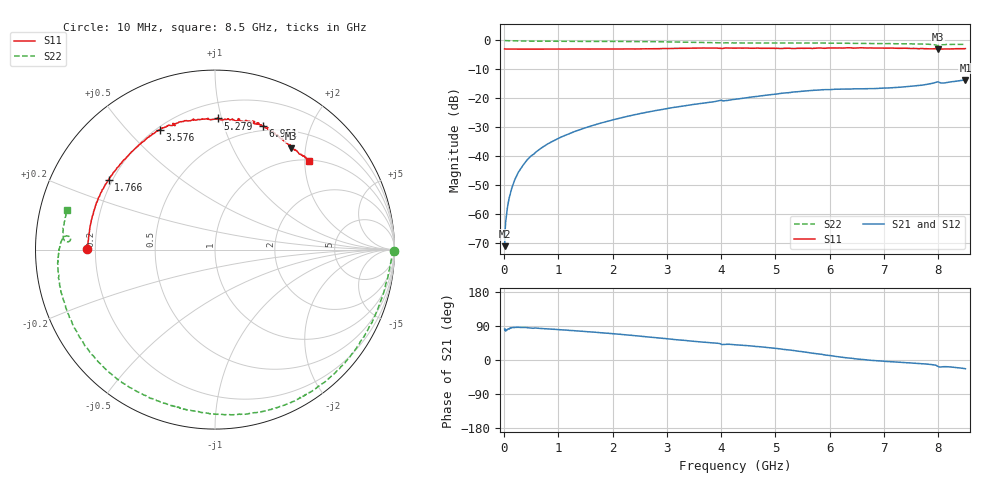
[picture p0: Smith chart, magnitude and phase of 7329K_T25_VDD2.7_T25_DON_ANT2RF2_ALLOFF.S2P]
!Agilent Technologies,E5071C,MY46417908,A.11.23
!Date: Mon Aug 31 18:03:31 2020
!Data & Calibration Information:
!Freq	S11:SOLT2(ON)	S21:SOLT2(ON)	S12:SOLT2(ON)	S22:SOLT2(ON)
!PortZ  Port1:50+j0  Port2:50+j0
!Above PortZ is port z conversion or system Z0 setting when saving the data.
!When reading, reference impedance value at option line is always used.
# Hz S dB R 50
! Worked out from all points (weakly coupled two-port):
!   1601 points, 10 MHz to 8.5 GHz, reference 50 ohm
!   highest |S21| = -13.61 dB at 8.5 GHz (marker M1); lowest = -71.0 dB at 10 MHz (marker M2)
!   lowest |S11| = -3.0 dB at 8.001 GHz (marker M3), VSWR 5.81, Z = 38.5 + j86.8 ohm
!   |S11| at or under -10 dB: nowhere
!   |S22| runs from -1.9 to 0.0 dB; largest |S21 - S12| = 0.003
!   S11 on the Smith chart (normalised r, x): 10 MHz: 0.17, +0.00; 1.766 GHz: 0.18, +0.29; 3.576 GHz: 0.21, +0.62; 5.279 GHz: 0.31, +0.97; 6.951 GHz: 0.45, +1.36; 8.5 GHz: 1.01, +2.10
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1e7  -2.95 179.8  -70.96 81.3  -70.53 82.9  -0.02 -0.4
6.836875e7  -2.99 178.5  -56.87 80.8  -57.05 80.9  -0.11 -2.0
1.214312e8  -2.99 177.3  -52.25 84.5  -52.21 84.3  -0.14 -3.3
2.169438e8  -3.01 175.3  -47.32 85.9  -47.27 86.3  -0.18 -5.3
3.389875e8  -3.01 173.0  -43.32 85.9  -43.29 86.2  -0.22 -8.1
4.822562e8  -3.01 170.1  -40.14 84.3  -40.15 84.5  -0.26 -11.4
7.634875e8  -3.00 164.8  -36.19 82.5  -36.19 82.5  -0.30 -17.7
1.426769e9  -2.98 152.8  -30.60 75.9  -30.58 75.9  -0.36 -33.4
1.766369e9  -2.98 146.6  -28.60 72.2  -28.59 72.2  -0.36 -41.4
2.843538e9  -2.85 126.1  -24.04 58.3  -24.04 58.2  -0.46 -67.0
3.5758e9  -2.66 114.8  -21.89 48.2  -21.88 48.3  -0.70 -86.0
4.255e9  -2.64 105.7  -20.33 40.2  -20.33 40.2  -0.88 -101.8
4.828075e9  -2.75 96.3  -18.90 33.2  -18.89 33.2  -0.90 -114.1
5.279106e9  -2.72 88.8  -17.96 26.2  -17.94 26.4  -0.89 -125.5
5.671769e9  -2.77 81.2  -17.25 18.3  -17.22 18.6  -0.91 -137.4
6.276681e9  -2.63 73.1  -16.78 6.4  -16.83 6.6  -0.99 -157.5
6.950575e9  -2.62 68.9  -16.53 -2.6  -16.58 -2.6  -1.10 -173.1
7.088538e9  -2.67 66.3  -16.40 -4.3  -16.44 -4.7  -1.11 -175.1
7.77835e9  -2.84 57.6  -15.20 -10.6  -15.23 -10.6  -1.30 178.0
8.001212e9  -3.02 53.1  -14.33 -17.4  -14.37 -17.4  -1.86 175.9
8.155094e9  -2.93 50.5  -14.54 -17.5  -14.57 -17.5  -1.40 174.3
8.5e9  -2.83 43.4  -13.61 -23.0  -13.68 -23.5  -1.37 165.0
